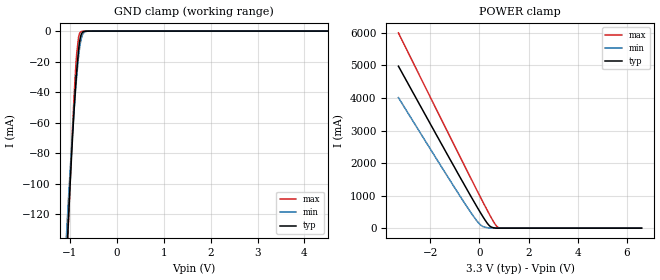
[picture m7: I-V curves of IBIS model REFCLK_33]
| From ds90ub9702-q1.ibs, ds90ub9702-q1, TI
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| REFCLK_3p3 Model
[Model]   REFCLK_33
Model_type   Input
Vinl = 0.8
Vinh = 2
|   typ   min   max
C_comp   1.157818pF   1.269522pF   1.055942pF
[Voltage Range]   3.3   3   3.6
[Temperature Range]   27   105   -40
[Power Clamp Reference]   3.3   3   3.6
[GND Clamp Reference]   0   0   0
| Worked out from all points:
|   GND clamp passes 1 mA (typ) near -0.74 V on its own axis
[GND Clamp]
|   Voltage   I(typ)   I(min)   I(max)
-3.3V     -1.861A    -1.697A    -2.01A
-1.073V   -152.4mA   -134.5mA   -157.6mA
-1.043V   -132.4mA   -117.7mA   -135mA
-1.033V   -125.8mA   -112.3mA   -127.6mA
-943.8mV  -70.59mA   -67.34mA   -64.28mA
-874.5mV  -35mA      -37.43mA   -23.89mA
-854.7mV  -26.49mA   -29.94mA   -15.25mA
-815.1mV  -12.57mA   -17.01mA   -4.163mA
-755.7mV  -2.128mA   -4.813mA   -295.1uA
-696.3mV  -233.6uA   -898.6uA   -33.49uA
-557.7mV  -12.56uA   -23.62uA   -13.99uA
6.6V      0A         0A         0A
[POWER Clamp]
|   Voltage   I(typ)   I(min)   I(max)
-3.3V     4.978A     4.012A     6.001A
-1.241V   2.172A     1.518A     2.871A
-537.9mV  1.228A     691.8mA    1.812A
-122.1mV  681.7mA    239.9mA    1.191A
16.5mV    504.9mA    118mA      985.8mA
125.4mV   370mA      55.66mA    825.9mA
382.8mV   92.01mA    7.414mA    455.7mA
491.7mV   30.59mA    865.2uA    305.5mA
630.3mV   4.936mA    56.22uA    130.3mA
729.3mV   305.4uA    41.79uA    38.91mA
917.4mV   50.14uA    37.74uA    226.6uA
6.6V      0A         0A         0A
